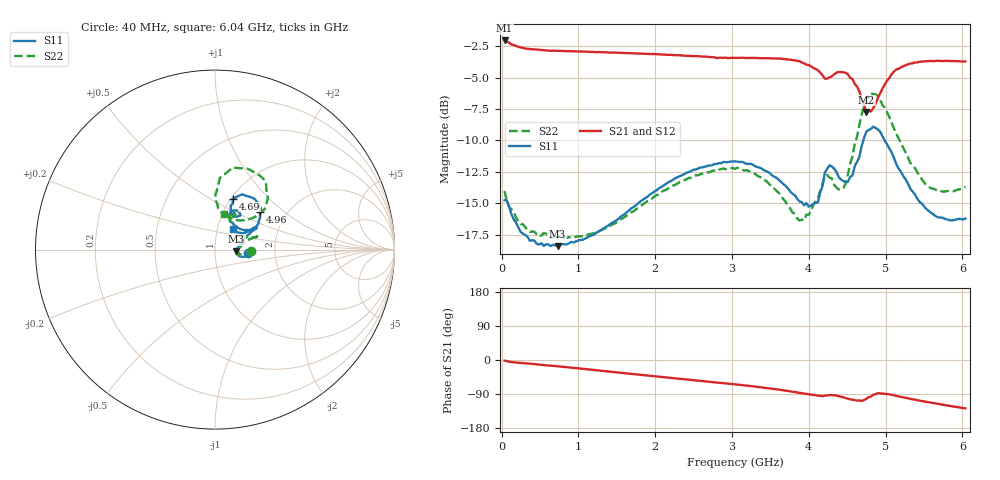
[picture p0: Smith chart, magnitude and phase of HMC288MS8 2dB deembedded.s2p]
!Hittite Microwave Corporation
!12 Elizabeth Drive
!Chelmsford, MA 01824
!Tel: 978-250-3343
!Fax: 978-250-3373
!Device: HMC288MS8, 0.7-3.7 GHz GaAs IC 3-bit Digital Attenuator in 8-lead Grounded Base surface Mount Plastic Package
!Misc:  2dB state, room
# GHZ S DB R 50.0
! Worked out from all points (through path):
!   201 points, 40 MHz to 6.04 GHz, reference 50 ohm
!   highest |S21| = -2.05 dB at 40 MHz (marker M1); lowest = -7.7 dB at 4.75 GHz (marker M2)
!   group delay of S21, straight-line fit = 55.5 ps
!   lowest |S11| = -18.4 dB at 730 MHz (marker M3), VSWR 1.27, Z = 63.6 - j1.21 ohm
!   |S11| at or under -10 dB: start of sweep to 4.711 GHz; 4.987 GHz to end of sweep
!   |S22| runs from -17.8 to -6.3 dB; largest |S21 - S12| = 0.0081
!   S11 on the Smith chart (normalised r, x): 40 MHz: 1.44, -0.05; 4.69 GHz: 1.02, +0.64; 4.96 GHz: 1.48, +0.70; 6.04 GHz: 1.19, +0.28
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0.04  -14.76 -5.4  -2.05 -1.6  -2.07 -1.4  -14.03 -1.8
0.1  -15.30 -13.4  -2.24 -4.7  -2.24 -4.5  -15.31 -10.1
0.34  -17.69 -13.4  -2.71 -9.2  -2.70 -9.3  -17.19 -11.3
0.73  -18.43 -4.5  -2.87 -16.5  -2.88 -16.6  -17.71 -6.6
1.06  -17.91 4.4  -2.93 -23.3  -2.93 -23.4  -17.64 -0.3
2.05  -13.81 24.2  -3.16 -44.0  -3.15 -44.2  -14.29 16.2
3.04  -11.69 27.7  -3.44 -64.3  -3.42 -64.4  -12.26 17.3
3.46  -12.48 28.2  -3.46 -74.0  -3.45 -74.1  -13.31 17.9
3.88  -14.87 39.0  -3.71 -86.6  -3.69 -86.8  -16.38 38.9
4.06  -15.07 55.2  -4.24 -92.2  -4.21 -92.5  -15.15 60.5
4.18  -13.64 68.3  -4.82 -95.5  -4.81 -95.6  -13.44 67.2
4.27  -11.99 59.7  -4.99 -92.4  -4.96 -92.5  -12.96 59.3
4.45  -13.24 57.2  -4.58 -98.2  -4.54 -98.4  -13.81 74.8
4.57  -12.78 67.5  -5.12 -104.7  -5.11 -105.0  -11.28 89.0
4.69  -10.44 70.6  -6.72 -108.0  -6.68 -108.2  -7.92 86.1
4.75  -9.30 63.9  -7.74 -102.7  -7.71 -103.5  -6.61 77.9
4.9  -9.14 44.2  -6.63 -87.7  -6.60 -88.3  -6.46 54.3
4.96  -9.68 39.7  -5.88 -88.7  -5.82 -89.0  -7.20 48.9
5.05  -10.65 33.6  -5.04 -90.9  -5.01 -90.9  -8.13 42.6
5.23  -12.84 28.5  -4.09 -98.6  -4.07 -98.8  -10.58 39.0
5.53  -15.46 33.8  -3.71 -110.3  -3.70 -110.5  -13.57 50.8
6.04  -16.22 48.9  -3.72 -127.8  -3.72 -127.9  -13.69 75.6
